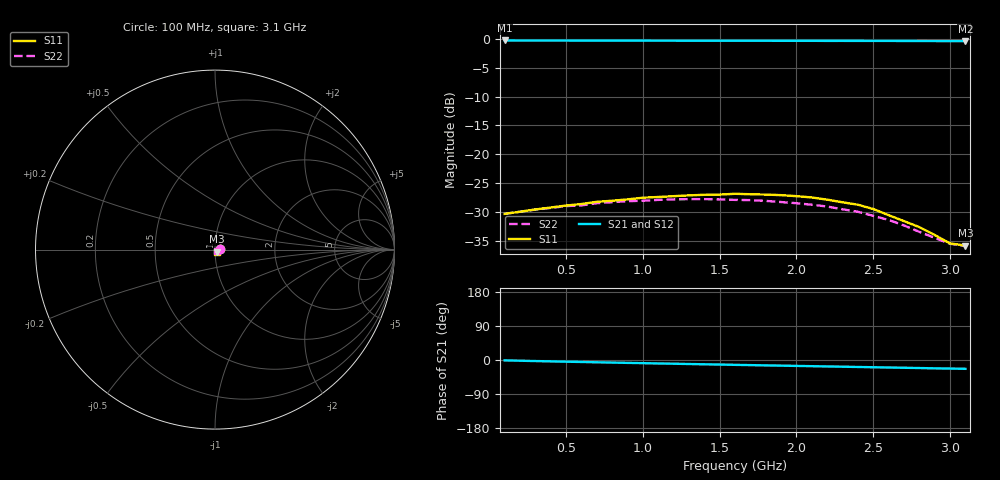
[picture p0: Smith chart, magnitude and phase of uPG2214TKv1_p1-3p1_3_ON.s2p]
! NEC Compound Semiconductor Devices Ltd.
! 4.February 2005
! uPG2214TK
! Vcont1=0v Vcont2=3.0v / IN-OUT1 ( ON )
! OUT2:50ohm termination
#  GHz  S  MA  R  50
!  f  S11  S21  S12  S22
!  GHz  MAG  ANG  MAG  ANG  MAG  ANG  MAG  ANG
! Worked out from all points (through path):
!   31 points, 100 MHz to 3.1 GHz, reference 50 ohm
!   highest |S21| = -0.26 dB at 100 MHz (marker M1); lowest = -0.4 dB at 3.1 GHz (marker M2)
!   group delay of S21, straight-line fit = 20.4 ps
!   lowest |S11| = -35.8 dB at 3.1 GHz (marker M3), VSWR 1.03, Z = 51 - j1.26 ohm
!   |S11| at or under -10 dB: start of sweep to end of sweep
!   |S22| runs from -35.9 to -27.8 dB; largest |S21 - S12| = 0.0022
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0.1  0.0305 7.0  0.9706 -1.0  0.9706 -1.0  0.0305 7.3
0.3  0.0333 15.6  0.9691 -2.8  0.9689 -2.8  0.0332 16.3
0.5  0.036 21.0  0.9684 -4.5  0.968 -4.4  0.0356 22.5
0.6  0.0371 24.4  0.9674 -5.2  0.968 -5.2  0.0361 25.5
0.7  0.0388 24.7  0.9675 -6.0  0.9671 -6.0  0.0377 27.1
0.9  0.0407 26.8  0.9672 -7.6  0.9663 -7.6  0.0393 30.9
1  0.0421 27.8  0.9664 -8.3  0.9662 -8.3  0.0396 32.9
1.1  0.0427 27.5  0.966 -9.1  0.9661 -9.1  0.0403 33.8
1.3  0.0441 27.5  0.9653 -10.6  0.9656 -10.6  0.0409 36.3
1.6  0.0455 26.6  0.9646 -12.8  0.9645 -12.8  0.0403 38.5
1.8  0.0448 25.2  0.9645 -14.2  0.9642 -14.2  0.0395 39.5
1.9  0.0443 24.3  0.9637 -14.9  0.9643 -14.9  0.0386 39.4
2.1  0.0423 22.3  0.9632 -16.3  0.9629 -16.3  0.0366 38.7
2.2  0.0405 20.9  0.9624 -17.0  0.9629 -17.0  0.0353 37.8
2.4  0.0366 21.3  0.9621 -18.4  0.9621 -18.4  0.0318 30.7
2.5  0.0336 14.3  0.9615 -19.1  0.9616 -19.1  0.0293 31.8
2.6  0.0297 10.8  0.9612 -19.8  0.9606 -19.8  0.027 27.9
2.7  0.0264 7.1  0.9609 -20.5  0.9601 -20.5  0.0242 22.3
2.8  0.0234 -0.7  0.9601 -21.2  0.9602 -21.1  0.0213 14.9
2.9  0.02 -13.3  0.9588 -22.0  0.9602 -21.9  0.0189 4.1
3  0.0169 -29.6  0.9582 -22.6  0.9598 -22.6  0.0168 -11.4
3.1  0.0162 -49.7  0.9578 -23.3  0.9583 -23.3  0.016 -30.7
